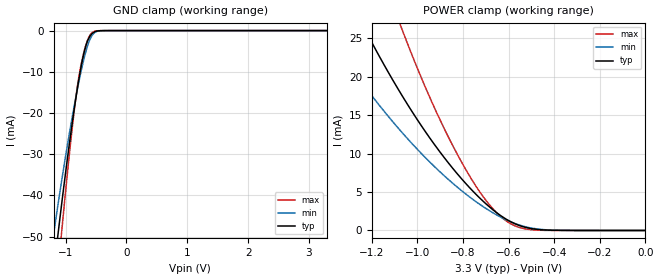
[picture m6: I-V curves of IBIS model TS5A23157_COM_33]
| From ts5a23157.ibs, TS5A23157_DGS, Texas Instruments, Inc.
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[Model]   TS5A23157_COM_33
Model_type  Terminator
| variable   typ   min   max
C_comp   16.01pF   11.65pF   17.63pF
| C_tri-state   16.01pF   11.65pF   17.63pF
[Temperature Range]   40   100   -40
| Ambient temperature   25   85   -40
[Voltage range]   3.3   3   3.6
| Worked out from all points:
|   GND clamp passes 1 mA (typ) near -0.58 V on its own axis
|   POWER clamp passes 1 mA (typ) near -0.58 V on its own axis
[GND Clamp]
| TS5A23157_COM_33
|   Voltage   I(typ)   I(min)   I(max)
-3.3V     -387.3mA   -317.3mA   -463.6mA
-1.205V   -59.4mA    -50.02mA   -71.06mA
-1.17V    -54.91mA   -46.51mA   -65.33mA
-1.12V    -48.63mA   -41.59mA   -57.28mA
-1.075V   -43.12mA   -37.27mA   -50.19mA
-1.045V   -39.53mA   -34.45mA   -45.56mA
-880mV    -21.14mA   -19.95mA   -22.01mA
-785mV    -12.01mA   -12.57mA   -11.39mA
-665mV    -3.565mA   -4.942mA   -3.368mA
-545mV    -485.6uA   -768.5uA   -302.2uA
-395mV    -12.13uA   -20.23uA   -2.239uA
3.3V      3.512nA    3.603uA    3.372nA
[POWER Clamp]
| TS5A23157_COM_33
|   Voltage   I(typ)   I(min)   I(max)
-3.3V     222.3mA    162.7mA    327.6mA
-1.415V   37.5mA     26.6mA     57.95mA
-1.39V    35.87mA    25.47mA    55.38mA
-1.23V    26.14mA    18.7mA     39.91mA
-1.065V   17.43mA    12.66mA    25.96mA
-945mV    12mA       8.88mA     17.26mA
-825mV    7.365mA    5.632mA    9.905mA
-730mV    4.315mA    3.468mA    5.163mA
-630mV    1.83mA     1.665mA    1.683mA
-570mV    842.5uA    880.8uA    568.1uA
-500mV    239.5uA    309.2uA    93.86uA
-48.03fV  3.512nA    4.045nA    3.688nA
